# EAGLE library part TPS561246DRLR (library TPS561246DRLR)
Switching Voltage Regulators 4.2V to 17V input voltage, 1A, 1.2MHz synchronous buck converter in SOT563 with FCCM mode Source: Datasheet
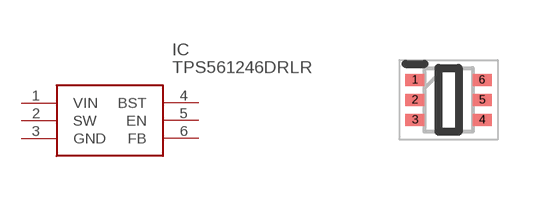
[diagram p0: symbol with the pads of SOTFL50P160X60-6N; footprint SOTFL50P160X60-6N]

Designator prefix IC

## TPS561246DRLR (Description: Switching Voltage Regulators 4.2V to 17V input voltage, 1A, 1.2MHz synchronous buck converter in SOT563 with FCCM mode; Height: 0.6mm; Manufacturer_Name: Texas Instruments; Manufacturer_Part_Number: TPS561246DRLR; Mouser_Part_Number: 595-TPS561246DRLR; Mouser_Price-Stock: https://www.mouser.co.uk/ProductDetail/Texas-Instruments/TPS561246DRLR?qs=IKkN%2F947nfBlLn983Qr7Pw%3D%3D)  [SOTFL50P160X60-6N]
1  VIN
2  SW
3  GND
4  BST
5  EN
6  FB

## Footprint SOTFL50P160X60-6N (pad centres in mm)
DRL0006A
smd 0.475 x 0.3: 1 -0.838,0.5; 2 -0.838,0; 3 -0.838,-0.5; 4 0.838,-0.5; 5 0.838,0; 6 0.838,0.5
